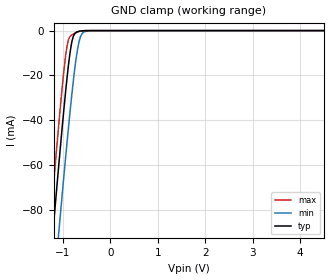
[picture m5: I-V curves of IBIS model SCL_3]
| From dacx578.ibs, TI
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|   SCL Model 3.3V MODEL
[Model] SCL_3
Model_type   Input
Vinl = 0.99
Vinh = 2.31
|   typ   min   max
|   (Nom PVT)   (Fast PVT)  (Slow PVT)
C_comp   1.0699730e-12   9.0057260e-13   1.2474190e-12
|Where nom PVT is Nom process, 3.3V, 27C
|Fast PVT is Strong Process, 3.6V, -40C
|Slow PVT is Weak Process,   3.0V, 125C
[Voltage Range]   3.3   3   3.6
[Temperature Range]   27   125   -40
|Junction temperatures are used for [Temperature Range]
[Power Clamp Reference]   3.3   3   3.6
[GND Clamp Reference]   0   0   0
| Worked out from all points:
|   GND clamp passes 1 mA (typ) near -0.73 V on its own axis
[GND Clamp]
|   Voltage   I(typ)   I(min)   I(max)
-3.3V     -634.1mA   -654.9mA   -622.8mA
-1.284V   -107.8mA   -137.5mA   -90.06mA
-1.218V   -91.26mA   -121.1mA   -73.27mA
-1.082V   -58.27mA   -88.4mA    -40.11mA
-940.9mV  -26.39mA   -55.69mA   -10.56mA
-885.7mV  -15.55mA   -43.57mA   -4.206mA
-821.1mV  -5.847mA   -29.98mA   -2.063mA
-776.7mV  -2.315mA   -21.4mA    -1.462mA
-702.8mV  -562.4uA   -9.717mA   -716.3uA
-600.2mV  -126.1uA   -1.395mA   -192.4uA
-410.8mV  -14.75uA   -15.71uA   -22.18uA
6.59V     0A         0A         0A
[POWER Clamp]
|   SCR cell for ESD function. Effects occurr above VDD x 2
|   Voltage   I(typ)   I(min)   I(max)
-3.3V     0A         0A         0A
0V        0A         0A         0A
6.6V      0A         0A         0A
